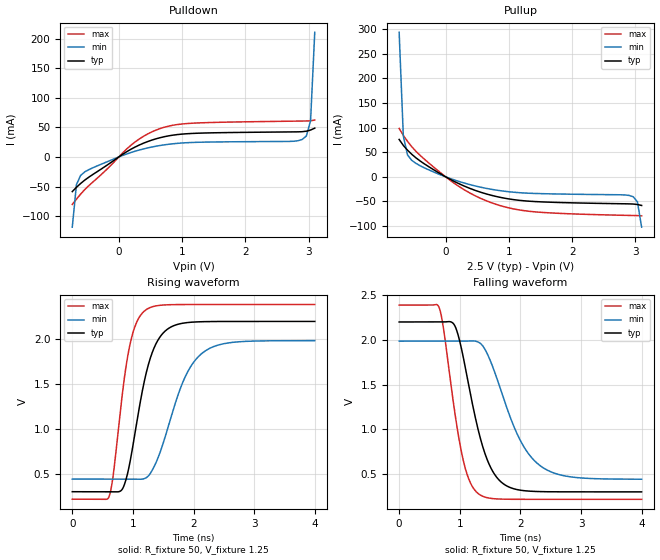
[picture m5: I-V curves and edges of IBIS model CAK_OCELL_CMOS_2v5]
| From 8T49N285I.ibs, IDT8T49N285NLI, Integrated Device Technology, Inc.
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[Model] CAK_OCELL_CMOS_2v5
Model_type   Output
Polarity   Non-Inverting
|   typ   min   max
C_comp   2pF   1.5pF   2.5pF
Vmeas = 1.25V
Rref = 50
Cref = 0
Vref = 1.25V
|   typ   min   max
[Voltage range]   2.5V   2.375V   2.625V
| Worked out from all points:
|   slope of the pulldown table from 0 to 0.375 V, typ, clamps not added: 16.6 ohm
|   slope of the pullup table from 0 to 0.375 V, typ, clamps not added: 16.3 ohm
|   rising waveform, R_fixture 50, V_fixture 1.25: 20-80 % time 336ps typ, 482ps min, 251ps max; typ from 0.3 V to 2.2 V
|   falling waveform, R_fixture 50, V_fixture 1.25: 20-80 % time 388ps typ, 553ps min, 290ps max; typ from 2.2 V to 0.3 V
[Pulldown]
|Voltage   I (typ)   I (min)   I (max)
|Note, modeling breaks down at 250mA and above.  This is well beyond the functional   |
|operating range of the device.  Should this scenario occur, catastrophic failure and   |
|possible damage to the device and/or board is of higher concern than the I-V curve   |
|behavior.  The IBIS checker will flag currents in excess of 10A with warnings.  Lines   |
|with currents in excess of 0.35 A have been commented out.  The points still remain|
|available to the user if the user desires to use them.   |
|-2.20000e+00   -1.46959e+01   -1.21350e+01   -1.76442e+01
|-1.90000e+00   -1.13595e+01   -9.63506e+00   -1.33803e+01
|-1.60000e+00   -8.02318e+00   -7.13538e+00   -9.11662e+00
|-1.30000e+00   -4.68697e+00   -4.63585e+00   -4.85419e+00
|-1.00000e+00   -1.35106e+00   -2.13641e+00   -5.91093e-01
|-9.99000e-01   -1.33995e+00   -2.12808e+00   -5.76880e-01
|-9.32920e-01   -6.05266e-01   -1.57759e+00   -1.28741e-01
|-8.66839e-01   -1.30215e-01   -1.02717e+00   -9.77767e-02
|-8.00759e-01   -6.99070e-02   -4.76818e-01   -8.89127e-02
-734.7mV  -58.45mA   -118.5mA   -80.18mA
-668.6mV  -51.17mA   -46.66mA   -71.18mA
-602.5mV  -44.74mA   -31.05mA   -62.69mA
-470.4mV  -33.87mA   -21.19mA   -48.15mA
58.29mV   4.327mA    2.464mA    6.617mA
454.8mV   25.98mA    15.27mA    38.76mA
851.3mV   36.81mA    22.26mA    53.55mA
1.38V     40.58mA    25.15mA    58.02mA
2.9V      42.73mA    29.61mA    60.73mA
2.966V    43.59mA    35.53mA    60.85mA
3.032V    45.53mA    61.23mA    61.17mA
3.098V    48.7mA     210.6mA    62.39mA
| 3.16407e+00   5.31861e-02   8.56282e-01   6.50885e-02
| 3.23015e+00   5.96810e-02   1.79353e+00   6.93284e-02
| 3.29623e+00   7.66643e-02   2.73471e+00   7.51228e-02
| 3.36231e+00   2.18225e-01   3.67600e+00   8.23322e-02
| 3.42839e+00   1.12672e+00   4.61744e+00   8.96971e-02
| 3.49447e+00   2.38353e+00   5.55905e+00   9.89240e-02
| 3.56055e+00   3.64056e+00   6.50082e+00   1.82013e-01
| 3.62663e+00   4.89783e+00   7.44276e+00   1.20124e+00
| 3.69271e+00   6.15534e+00   8.38487e+00   2.80877e+00
| 3.75879e+00   7.41309e+00   9.32716e+00   4.41662e+00
| 3.82487e+00   8.67110e+00   1.02696e+01   6.02477e+00
| 3.89095e+00   9.92934e+00   1.12123e+01   7.63323e+00
| 3.95703e+00   1.11878e+01   1.21551e+01   9.24199e+00
| 4.02311e+00   1.24466e+01   1.30981e+01   1.08511e+01
| 4.08920e+00   1.37056e+01   1.40413e+01   1.24604e+01
| 4.15528e+00   1.49648e+01   1.49847e+01   1.40701e+01
| 4.22136e+00   1.62243e+01   1.59283e+01   1.56800e+01
| 4.28744e+00   1.74840e+01   1.68720e+01   1.72902e+01
| 4.35352e+00   1.87440e+01   1.78160e+01   1.89007e+01
| 4.41960e+00   2.00042e+01   1.87602e+01   2.05115e+01
| 4.48568e+00   2.12646e+01   1.97045e+01   2.21227e+01
| 4.55176e+00   2.25253e+01   2.06491e+01   2.37342e+01
| 4.61784e+00   2.37863e+01   2.15939e+01   2.53461e+01
| 4.68392e+00   2.50475e+01   2.25388e+01   2.69583e+01
| 4.75000e+00   2.63089e+01   2.34840e+01   2.85708e+01
| 4.75100e+00   2.63280e+01   2.34983e+01   2.85952e+01
| 4.80080e+00   2.72789e+01   2.42108e+01   2.98106e+01
| 4.85060e+00   2.82299e+01   2.49234e+01   3.10263e+01
| 4.90040e+00   2.91811e+01   2.56362e+01   3.22421e+01
| 4.95020e+00   3.01324e+01   2.63490e+01   3.34581e+01
| 5.00000e+00   3.10839e+01   2.70620e+01   3.46743e+01
[Pullup]
|Voltage   I (typ)   I (min)   I (max)
|Note, modeling breaks down at 250mA and above.  This is well beyond the functional   |
|operating range of the device.  Should this scenario occur, catastrophic failure and   |
|possible damage to the device and/or board is of higher concern than the I-V curve   |
|behavior.  The IBIS checker will flag currents in excess of 10A with warnings.  Lines   |
|with currents in excess of 0.35 A have been commented out.  The points still remain|
|available to the user if the user desires to use them.   |
|-2.20000e+00   2.54368e+01   2.10499e+01   3.04934e+01
|-1.90000e+00   1.97039e+01   1.67545e+01   2.31657e+01
|-1.60000e+00   1.39741e+01   1.24622e+01   1.58417e+01
|-1.30000e+00   8.24739e+00   8.17256e+00   8.52039e+00
|-1.00000e+00   2.52317e+00   3.88510e+00   1.20144e+00
|-9.99000e-01   2.50409e+00   3.87081e+00   1.17704e+00
|-9.32920e-01   1.24341e+00   2.92658e+00   2.07209e-01
|-8.66839e-01   2.72789e-01   1.98226e+00   1.28133e-01
|-8.00759e-01   1.00739e-01   1.03730e+00   1.13044e-01
-734.7mV  75.79mA    293mA      98.11mA
-668.6mV  63.64mA    82.61mA    84.02mA
-602.5mV  54.04mA    44.44mA    71.86mA
-536.4mV  45.8mA     33.49mA    61.25mA
-272.1mV  20.96mA    14.42mA    28.68mA
190.4mV   -12.75mA   -8.569mA   -17.85mA
520.9mV   -29.86mA   -20.14mA   -41.79mA
851.3mV   -41.34mA   -27.93mA   -57.97mA
1.446V    -50.4mA    -33.89mA   -71.42mA
2.9V      -54.87mA   -37.76mA   -78.3mA
3.032V    -56.14mA   -50.72mA   -78.7mA
3.098V    -58.11mA   -102.1mA   -79.22mA
| 3.16407e+00   -6.12362e-02   -3.89159e-01   -8.07508e-02
| 3.23015e+00   -6.56468e-02   -9.32725e-01   -8.38980e-02
| 3.29623e+00   -7.41383e-02   -1.48170e+00   -8.86088e-02
| 3.36231e+00   -1.24234e-01   -2.03086e+00   -9.45061e-02
| 3.42839e+00   -5.56732e-01   -2.58016e+00   -1.00802e-01
| 3.49447e+00   -1.28986e+00   -3.12957e+00   -1.07735e-01
| 3.56055e+00   -2.02321e+00   -3.67908e+00   -1.39910e-01
| 3.62663e+00   -2.75678e+00   -4.22867e+00   -6.20318e-01
| 3.69271e+00   -3.49053e+00   -4.77834e+00   -1.55812e+00
| 3.75879e+00   -4.22445e+00   -5.32808e+00   -2.49604e+00
| 3.82487e+00   -4.95850e+00   -5.87789e+00   -3.43407e+00
| 3.89095e+00   -5.69268e+00   -6.42776e+00   -4.37218e+00
| 3.95703e+00   -6.42695e+00   -6.97770e+00   -5.31039e+00
| 4.02311e+00   -7.16132e+00   -7.52770e+00   -6.24876e+00
| 4.08920e+00   -7.89577e+00   -8.07777e+00   -7.18732e+00
| 4.15528e+00   -8.63029e+00   -8.62789e+00   -8.12609e+00
| 4.22136e+00   -9.36489e+00   -9.17807e+00   -9.06502e+00
| 4.28744e+00   -1.00996e+01   -9.72830e+00   -1.00041e+01
| 4.35352e+00   -1.08343e+01   -1.02786e+01   -1.09433e+01
| 4.41960e+00   -1.15691e+01   -1.08289e+01   -1.18825e+01
| 4.48568e+00   -1.23039e+01   -1.13793e+01   -1.28218e+01
| 4.55176e+00   -1.30388e+01   -1.19298e+01   -1.37612e+01
| 4.61784e+00   -1.37738e+01   -1.24803e+01   -1.47007e+01
| 4.68392e+00   -1.45088e+01   -1.30308e+01   -1.56402e+01
| 4.75000e+00   -1.52438e+01   -1.35814e+01   -1.65798e+01
| 4.75100e+00   -1.52550e+01   -1.35898e+01   -1.65940e+01
| 4.80080e+00   -1.58090e+01   -1.40047e+01   -1.73022e+01
| 4.85060e+00   -1.63630e+01   -1.44198e+01   -1.80104e+01
| 4.90040e+00   -1.69171e+01   -1.48348e+01   -1.87186e+01
| 4.95020e+00   -1.74712e+01   -1.52499e+01   -1.94269e+01
| 5.00000e+00   -1.80253e+01   -1.56650e+01   -2.01352e+01
[Ramp]
|   typ   min   max
dV/dt_r   1.141/0.336n   0.928/0.482n   1.305/0.25n
dV/dt_f   1.143/0.388n   0.929/0.553n   1.308/0.291n
R_load =   50.0000
[Rising Waveform]
R_fixture = 50
V_fixture = 1.25   |Vcc_typ
V_fixture_min = 1.1875 |Vcc_min
V_fixture_max = 1.3125 |Vcc_max
C_fixture = 0.0p
| Time   typ   min   max
0s        300mV      441.1mV    216.5mV
608.9ps   300mV      441.1mV    248mV
680ps     300mV      441.1mV    509.3mV
817.8ps   321.2mV    441.1mV    1.346V
933.3ps   567.6mV    441.2mV    1.883V
1.2ns     1.569V     449.3mV    2.323V
1.516ns   2.083V     876mV      2.385V
1.84ns    2.183V     1.549V     2.39V
2.142ns   2.198V     1.846V     2.39V
4ns       2.201V     1.987V     2.39V
[Falling Waveform]
R_fixture = 50
V_fixture = 1.25   |Vcc_typ
V_fixture_min = 1.1875 |Vcc_min
V_fixture_max = 1.3125 |Vcc_max
C_fixture = 0.0p
| Time   typ   min   max
0s        2.201V     1.987V     2.39V
657.8ps   2.201V     1.987V     2.365V
733.3ps   2.201V     1.987V     2.121V
942.2ps   2.121V     1.987V     1.079V
1.111ns   1.623V     1.987V     516.3mV
1.302ns   998.7mV    1.977V     282.1mV
1.653ns   429mV      1.488V     219.7mV
1.978ns   321.2mV    903.6mV    216.7mV
2.293ns   303.5mV    610.6mV    216.5mV
4ns       300mV      441.5mV    216.5mV
